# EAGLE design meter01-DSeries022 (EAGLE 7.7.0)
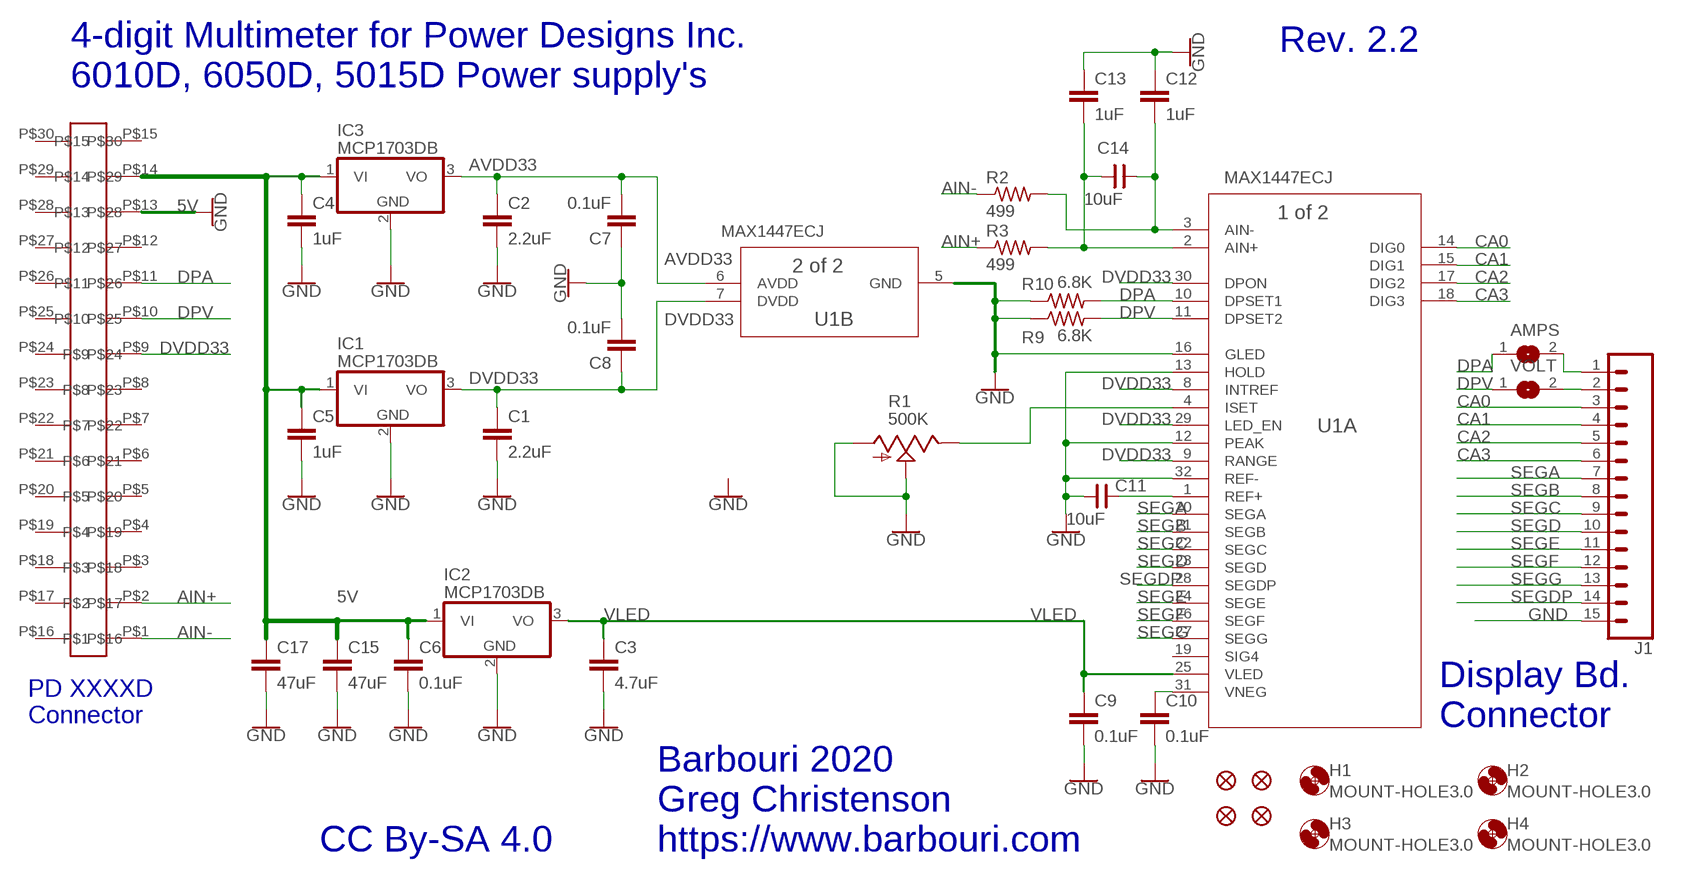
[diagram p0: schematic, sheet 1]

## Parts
AMPS  SJ  [SJ]
C1  2.2uF  2.2UF-0805-25V-(+80/-20%)  [0805]
C2  2.2uF  2.2UF-0805-25V-(+80/-20%)  [0805]
C3  4.7uF  2.2UF-0805-25V-(+80/-20%)  [0805]
C4  1uF  0.1UF-0603-25V-5%  [0603]
C5  1uF  0.1UF-0603-25V-5%  [0603]
C6  0.1uF  0.1UF-0603-25V-5%  [0603]
C7  0.1uF  0.1UF-0603-25V-5%  [0603]
C8  0.1uF  0.1UF-0603-25V-5%  [0603]
C9  0.1uF  0.1UF-0603-25V-5%  [0603]
C10  0.1uF  0.1UF-0603-25V-5%  [0603]
C11  10uF  CNP-0805  [0805]
C12  1uF  0.1UF-0603-25V-5%  [0603]
C13  1uF  0.1UF-0603-25V-5%  [0603]
C14  10uF  CNP-0805  [0805]
C15  47uF  C-EUC1206  [C1206]
C17  47uF  C-EUC1206  [C1206]
FD1  FIDUCIALUFIDUCIAL  [FIDUCIAL-MICRO]
FD2  FIDUCIALUFIDUCIAL  [FIDUCIAL-MICRO]
FD3  FIDUCIALUFIDUCIAL  [FIDUCIAL-MICRO]
FD4  FIDUCIALUFIDUCIAL  [FIDUCIAL-MICRO]
H1  MOUNT-HOLE3.0  [3,0]
H2  MOUNT-HOLE3.0  [3,0]
H3  MOUNT-HOLE3.0  [3,0]
H4  MOUNT-HOLE3.0  [3,0]
IC1  MCP1703DB  [SOT223]
IC2  MCP1703DB  [SOT223]
IC3  MCP1703DB  [SOT223]
J1  CONN_15LOCK  [1X15_LOCK]
R1  500K  TRIM_US-SM-42/43W  [SM-42/43W]
R2  499  R-US_M1206  [M1206]
R3  499  R-US_M1206  [M1206]
R9  6.8K  R-US_R0805  [R0805]
R10  6.8K  R-US_R0805  [R0805]
U1  MAX1447ECJ  MAX1447ECJ+21-0054G_32-L  [21-0054G_32-L]
U$2  EDGECARD15  [EDGECARD15]
VOLT  SJ  [SJ]

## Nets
5V: C4.1 C5.1 C6.1 C15.1 C17.1 IC1.1(VI) IC2.1(VI) IC3.1(VI) U$2.P$14
AIN+: R3.1 U$2.P$2
AIN-: R2.1 U$2.P$1
AVDD33: C2.1 C7.2 IC3.3(VO) U1.6(B:AVDD)
CA0: J1.3 U1.14(A:DIG0)
CA1: J1.4 U1.15(A:DIG1)
CA2: J1.5 U1.17(A:DIG2)
CA3: J1.6 U1.18(A:DIG3)
DPA: AMPS.1 R10.2 U1.10(A:DPSET1) U$2.P$11
DPV: R9.2 U1.11(A:DPSET2) U$2.P$10 VOLT.1
DVDD33: C1.1 C8.1 IC1.3(VO) U1.7(B:DVDD) U1.8(A:INTREF) U1.9(A:RANGE) U1.29(A:LED_EN) U1.30(A:DPON) U$2.P$9
GND: C1.2 C2.2 C3.2 C4.2 C5.2 C6.2 C7.1 C8.2 C9.2 C10.2 C11.1 C12.1 C13.1 C15.2 C17.2 IC1.2(GND) IC2.2(GND) IC3.2(GND) J1.15 R1.1(A) R1.2(S) R9.1 R10.1 U1.5(B:GND) U1.12(A:PEAK) U1.13(A:HOLD) U1.16(A:GLED) U1.32(A:REF-) U$2.P$13
N$1: C13.2 C14.1 R3.2 U1.2(A:AIN+)
N$2: C12.2 C14.2 R2.2 U1.3(A:AIN-)
N$5: AMPS.2 J1.1
N$6: J1.2 VOLT.2
N$7: R1.3(E) U1.4(A:ISET)
N$9: C10.1 U1.31(A:VNEG)
N$10: C11.2 U1.1(A:REF+)
SEGA: J1.7 U1.20(A:SEGA)
SEGB: J1.8 U1.21(A:SEGB)
SEGC: J1.9 U1.22(A:SEGC)
SEGD: J1.10 U1.23(A:SEGD)
SEGDP: J1.14 U1.28(A:SEGDP)
SEGE: J1.11 U1.24(A:SEGE)
SEGF: J1.12 U1.26(A:SEGF)
SEGG: J1.13 U1.27(A:SEGG)
VLED: C3.1 C9.1 IC2.3(VO) U1.25(A:VLED)
Unconnected: U1.19(A:SIG4) U$2.P$3 U$2.P$4 U$2.P$5 U$2.P$6 U$2.P$7 U$2.P$8 U$2.P$12 U$2.P$15 U$2.P$16 U$2.P$17 U$2.P$18 U$2.P$19 U$2.P$20 U$2.P$21 U$2.P$22 U$2.P$23 U$2.P$24 U$2.P$25 U$2.P$26 U$2.P$27 U$2.P$28 U$2.P$29 U$2.P$30

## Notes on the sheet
- Rev. 2.2
- 4-digit Multimeter for Power Designs Inc.
  6010D, 6050D, 5015D Power supply's
- PD XXXXD
  Connector
- Display Bd.
  Connector
- CC By-SA 4.0
- Barbouri 2020
  Greg Christenson
  https://www.barbouri.com

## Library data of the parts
AMPS VOLT = jumper:SJ: SMD solder JUMPER
C1 C2 = SparkFun-Capacitors:2.2UF: 2.2µF ceramic capacitors; PROD_ID: CAP-11624
C3 = SparkFun-Capacitors:2.2UF: 2.2µF ceramic capacitors; PROD_ID: CAP-11624; VALUE: 2.2uF
C4 C5 = SparkFun-Capacitors:0.1UF: 0.1µF ceramic capacitors; PROD_ID: CAP-08604; VALUE: 0.1uF
C6-C10 = SparkFun-Capacitors:0.1UF: 0.1µF ceramic capacitors; PROD_ID: CAP-08604
C11 = cap-master:CNP-: NON-POLARIZED CAP; DESC: 10µF ±10% 10V Ceramic Capacitor X7R 0805 (2012 Metric); MFG: AVX Corp; PN: 0805ZC106KAT4A
C12 C13 = SparkFun-Capacitors:0.1UF: 0.1µF ceramic capacitors; DESC: 1µF ±10% 16V Ceramic Capacitor X7R 0603 (1608 Metric); MFG: Vishay Vitramon; PN: VJ0603Y105KXJCW1BC; PROD_ID: CAP-08604; VALUE: 0.1uF
C14 = cap-master:CNP-: NON-POLARIZED CAP
C15 C17 = resistor:C-EU: CAPACITOR, European symbol; DESC: 47µF Molded Tantalum Capacitors 10V 1206 (3216 Metric) 1.5Ohm; MFG: AVX Corp; PN: TLJG476M010R1500
FD1-FD4 = SparkFun-Aesthetics:FIDUCIAL: Fiducial Alignment Points
H1-H4 = holes:MOUNT-HOLE: MOUNTING HOLE with drill center marker
IC1-IC3 = linear:MCP1703: 250 mA, 16V, Low Quiescent Current LDO Regulator Source: http://ww1.microchip.com/downloads/en/DeviceDoc/22049b.pdf
J1 = SparkFun-Connectors:CONN_15: Multi connection point. Often used as Generic Header-pin footprint for 0.1 inch spaced/style header connections On any of the 0.1 inch spaced packages, you can populate with these: Break Away Headers - Straight (PRT-00116) Break Away Male Headers - Right Angle (PRT-00553) Female Headers (PRT-00115)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
R1 = pot:TRIM_US-: POTENTIOMETER; DESC: 500 kOhms 0.25W, 1/4W J Lead Surf Mnt Trimmer Cermet 12 Turn Top Adj; MFG: Bourns Inc; PN: 3224W-1-504E
R2 R3 = resistor:R-US_: RESISTOR, American symbol; DESC: 499 Ohms ±0.1% 0.4W, 2/5W 1206 Non-Inductive Thin Film; MFG: Vishay Thin Film; PN: PTN1206Y4990BST1
R9 R10 = resistor:R-US_: RESISTOR, American symbol
U1 = MAX1447:MAX1447ECJ+; MANUFACTURER_PART_NUMBER: MAX1447ECJ+; VENDOR: Maxim Integrated Products
U$2 = User-Submitted:EDGECARD15: 15 pin edge card connector fingers 0.1" spacing 0.25" length. top and bottom layers 30 total pins

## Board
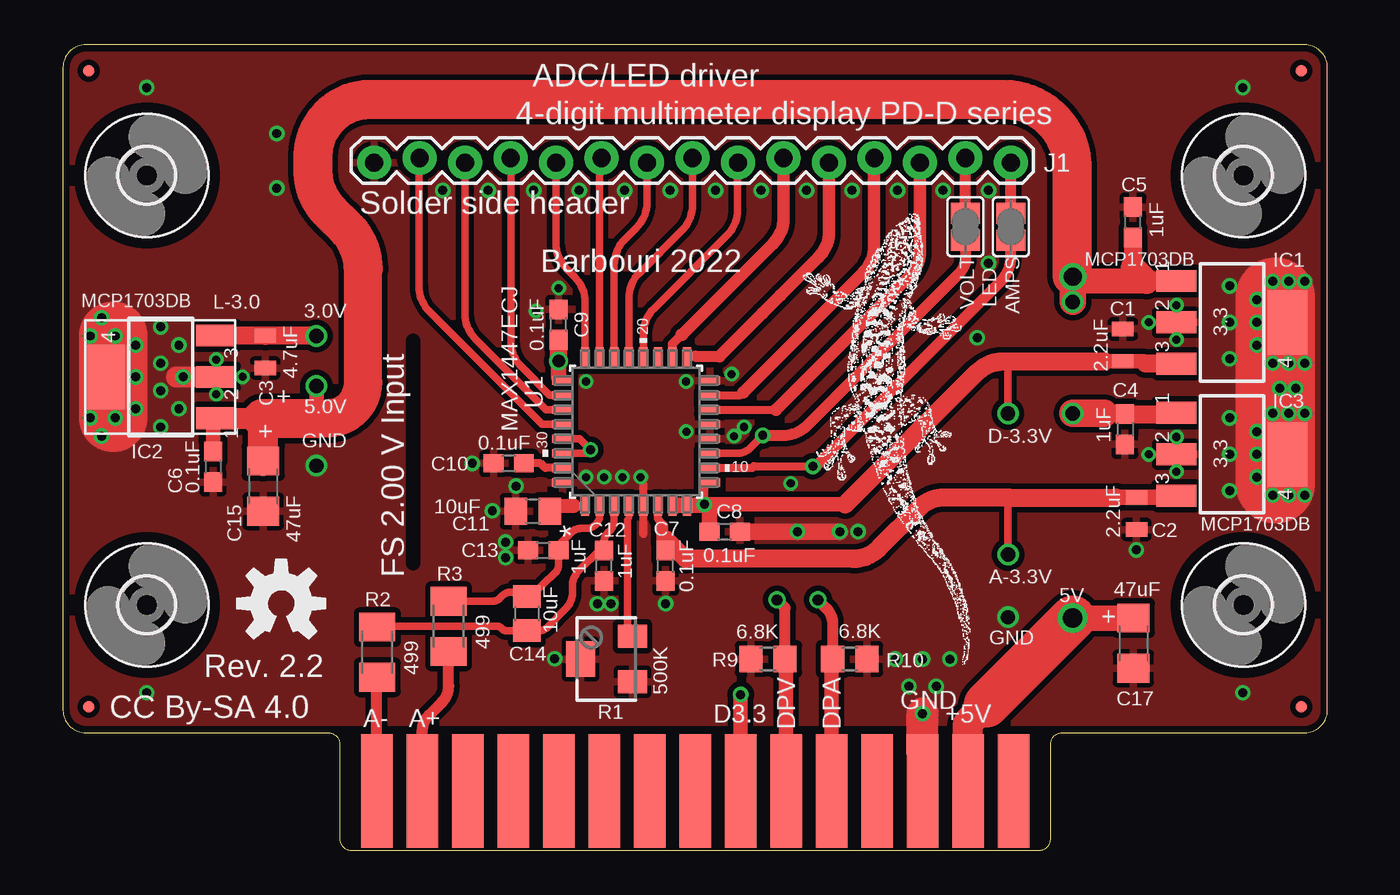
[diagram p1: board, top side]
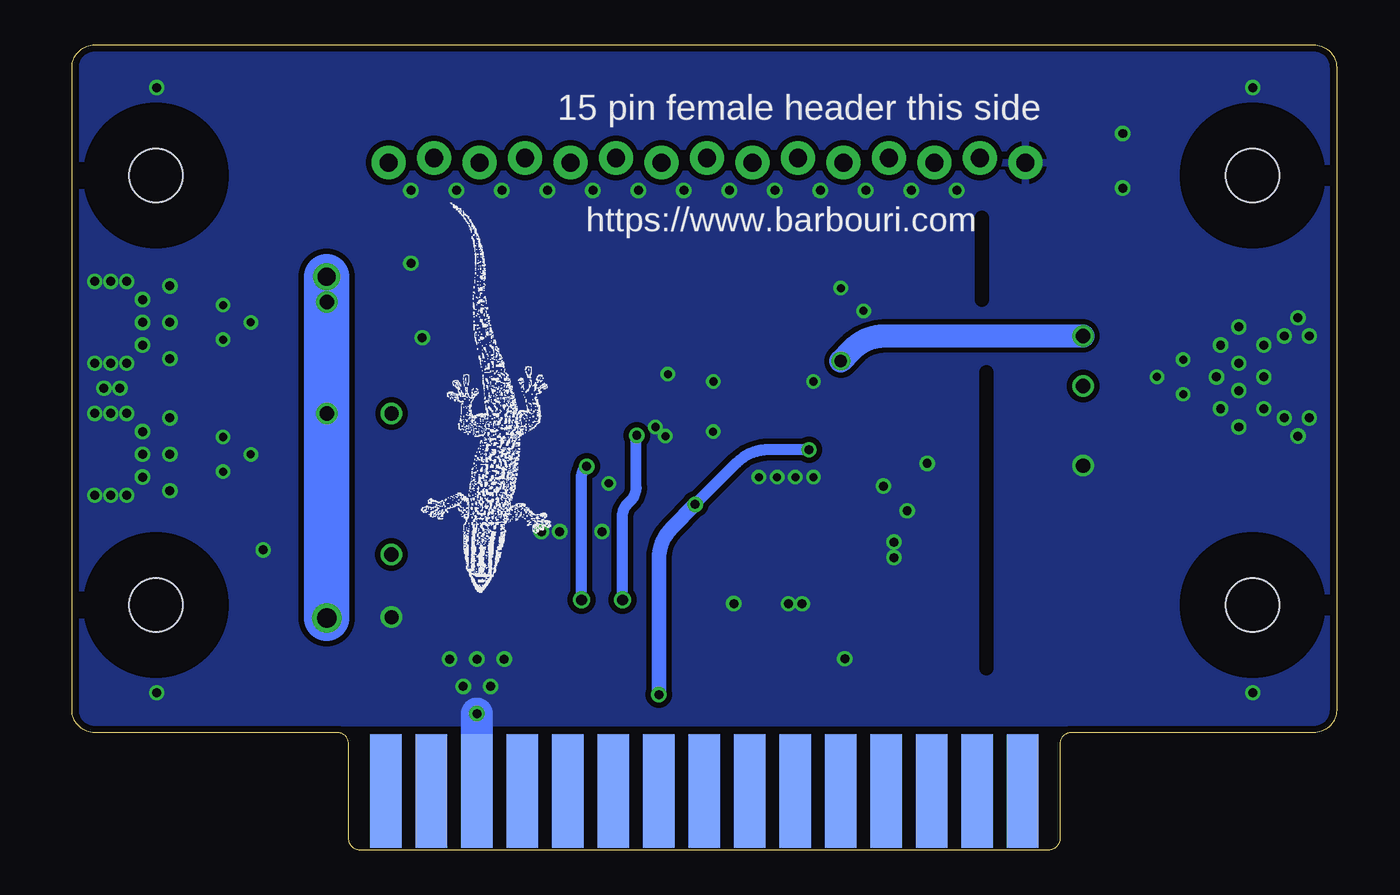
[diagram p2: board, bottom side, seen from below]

Size 70.61 x 44.96 mm. Coordinates in mm from the lower left corner, seen from the top.
Outline: 55.75,6.55 69.34,6.55 arc90 70.61,7.82 70.61,43.69 arc90 69.34,44.96 1.27,44.96 arc90 0,43.69 0,7.82 arc90 1.27,6.55 14.86,6.55 arc-90 15.44,5.92 15.44,0.64 arc90 16.13,0 54.48,0 arc90 55.17,0.64 55.17,5.92 arc-90 55.75,6.55
Copper layers (1*16): Top 0.0356mm / dielectric 1.5011mm / Bottom 0.0356mm
Design rules "oshpark-2layer *": minimum track width 16mil, minimum drill 9mil, track to track 12mil, track to pad 12mil, pad to pad 12mil, via to via 8mil, smd to smd 8mil, copper to edge 15mil, drill to drill 6mil, minimum pad ring 7mil, minimum via ring 7mil, stop-mask expansion 2.5mil, vias tented up to drill 20mil, thermal gap 10mil
tRestrict: 1 lines
bRestrict: 2 lines

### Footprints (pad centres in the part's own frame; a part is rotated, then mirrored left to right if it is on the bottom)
SJ = smd 1.168 x 1.6: 1 -0.762,0; 2 0.762,0
0805 = smd 0.8 x 1.2: 1 -0.9,0; 2 0.9,0
0603 = smd 1.1 x 1: 1 -0.85,0; 2 0.85,0
0805' = smd 1.27 x 1.524: 1 -0.953,0; 2 0.953,0
C1206 = smd 1.6 x 1.8: 1 -1.4,0; 2 1.4,0
FIDUCIAL-MICRO = smd 0.635 x 0.635: 1 0,0
3,0 = hole 3: 0,0
SOT223 = smd 1.219 x 2.235: 1 -2.311,-3.099; 2 0,-3.099; 3 2.311,-3.099 | smd 3.6 x 2.2: 4 0,3.099
1X15_LOCK = drill 1.016 pad 1.88: 1 0,0.127; 2 2.54,-0.127; 3 5.08,0.127; 4 7.62,-0.127; 5 10.16,0.127; 6 12.7,-0.127; 7 15.24,0.127; 8 17.78,-0.127; 9 20.32,0.127; 10 22.86,-0.127; 11 25.4,0.127; 12 27.94,-0.127; 13 30.48,0.127; 14 33.02,-0.127; 15 35.56,0.127
SM-42/43W = smd 1.3 x 1.6: 1 -1.27,-1.45; 3 1.27,-1.45 | smd 2 x 1.6: 2 0,1.45
M1206 = smd 1.6 x 2: 1 -1.4,0; 2 1.4,0
R0805 = smd 1.3 x 1.5: 1 -0.95,0; 2 0.95,0
21-0054G_32-L = smd 1.168 x 0.457: 1 -4.115,2.845; 2 -4.115,2.032; 3 -4.115,1.219; 4 -4.115,0.406; 5 -4.115,-0.406; 6 -4.115,-1.219; 7 -4.115,-2.032; 8 -4.115,-2.845; 17 4.115,-2.845; 18 4.115,-2.032; 19 4.115,-1.219; 20 4.115,-0.406; 21 4.115,0.406; 22 4.115,1.219; 23 4.115,2.032; 24 4.115,2.845 | smd 0.457 x 1.168: 9 -2.845,-4.115; 10 -2.032,-4.115; 11 -1.219,-4.115; 12 -0.406,-4.115; 13 0.406,-4.115; 14 1.219,-4.115; 15 2.032,-4.115; 16 2.845,-4.115; 25 2.845,4.115; 26 2.032,4.115; 27 1.219,4.115; 28 0.406,4.115; 29 -0.406,4.115; 30 -1.219,4.115; 31 -2.032,4.115; 32 -2.845,4.115
EDGECARD15 = smd 1.778 x 6.35: P$1 -17.78,3.302; P$2 -15.24,3.302; P$3 -12.7,3.302; P$4 -10.16,3.302; P$5 -7.62,3.302; P$6 -5.08,3.302; P$7 -2.54,3.302; P$8 0,3.302; P$9 2.54,3.302; P$10 5.08,3.302; P$11 7.62,3.302; P$12 10.16,3.302; P$13 12.7,3.302; P$14 15.24,3.302; P$15 17.78,3.302 | smd 1.778 x 6.35 bottom: P$16 -17.78,3.302; P$17 -15.24,3.302; P$18 -12.7,3.302; P$19 -10.16,3.302; P$20 -7.62,3.302; P$21 -5.08,3.302; P$22 -2.54,3.302; P$23 0,3.302; P$24 2.54,3.302; P$25 5.08,3.302; P$26 7.62,3.302; P$27 10.16,3.302; P$28 12.7,3.302; P$29 15.24,3.302; P$30 17.78,3.302

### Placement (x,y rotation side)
AMPS  52.93,34.8 90 top
C1  59.18,28.19 90 top
C2  59.94,18.8 270 top
C3  11.3,27.81 270 top
C4  59.31,23.5 270 top
C5  59.75,35.05 90 top
C6  8.38,21.4 270 top
C7  33.66,15.88 90 top
C8  36.96,17.78 0 top
C9  27.69,29.34 90 top
C10  24.89,21.59 180 top
C11  10uF  [0805']  26.24,18.92 0 top
C12  30.23,15.88 90 top
C13  26.82,16.74 0 top
C14  10uF  [0805']  25.91,13.21 270 top
C15  11.18,20.32 270 top
C17  59.78,11.56 270 top
FD1  69.16,8 90 top
FD2  1.45,8 90 top
FD3  69.16,43.51 90 top
FD4  1.45,43.51 90 top
H1  4.69,13.69 0 top
H2  65.93,13.69 0 top
H3  4.69,37.67 0 top
H4  65.93,37.67 0 top
IC1  65.28,29.46 270 top
IC2  5.46,26.42 90 top
IC3  65.28,22.1 270 top
J1  52.93,38.51 180 top
R1  30.35,10.67 90 top
R2  17.55,11.05 90 top
R3  21.54,12.5 90 top
R9  39.37,10.67 0 top
R10  43.94,10.67 180 top
U1  32,23.37 90 top
U$1  [OSHW-LOGO-M]  12.19,13.77 0 top
U$2  35.31,0 0 top
VOLT  50.39,34.8 90 top

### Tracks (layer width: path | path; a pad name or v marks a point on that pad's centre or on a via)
5V  (via drill 0.8, 1, 1.1)
  Top 0.61: 8.38,23.68 arc-45 IC2.1
  Top 0.813: 62.12,24.34 IC3.1 | v14.16,25.91 14.15,24.11 | C6.1 8.38,23.68
  Top 1.016: 62.12,24.34 C4.1 59.52,24.38 58.17,24.38 | IC1.1 60.54,31.77 | 60.54,31.77 60.52,31.75 | 60.54,31.77 60.48,31.77 | 59.77,32.49 59.77,34.19 C5.1
  Top 1.168: IC2.1 11.15,24.11
  Top 1.27: 56.45,31.75 v56.39,32 | v56.39,12.96 v56.39,12.95
  Top 1.397: 60.52,31.75 56.45,31.75 | 60.48,31.77 59.77,32.49
  Top 1.422: C17.1 v56.39,12.96
  Top 1.473: v56.39,30.61 v56.39,32
  Top 1.524: v56.39,24.38 58.17,24.38
  Top 1.676: U$2.P$14 50.55,7.11 51.56,8.13 | 14.15,24.11 14.2,24.11 | C15.1 11.18,24.04 arc45 11.15,24.11
  Top 1.93: 14.2,24.11 14.76,24.11 | 56.35,32.04 v56.39,32
  Top 2.134: 14.76,24.11 arc90 16.76,26.11 16.76,32.47
  Top 2.184: 11.15,24.11 14.15,24.11 | 16.76,32.47 arc45 15.83,34.71 14.9,35.65 arc-45 13.97,37.89 13.97,38.73 arc-90 17.14,41.91 52.54,41.91 arc-90 56.35,38.1 56.35,32.04
  Top 2.54: 51.56,8.13 v56.39,12.95
  Bottom 2.54: v56.39,12.95 v56.39,24.38 v56.39,32
AIN+
  Top 0.61: U$2.P$2 20.07,6.64 arc-45 20.44,7.54 21.17,8.26 arc45 21.54,9.16 R3.1
AIN-
  Top 0.61: U$2.P$1 17.53,9.12 R2.1
AVDD33  (via drill 0.8)
  Top 0.406: v52.78,16.51 52.76,16.54 52.76,19.63 52.78,19.63 52.83,19.68
  Top 0.457: 33.48,18.09 33.45,18.19 33.22,18.52 U1.6
  Top 0.61: 33.66,17.37 33.55,17.35 33.48,17.17
  Top 0.66: 33.48,17.17 33.48,18.09
  Top 0.813: 62.09,19.7 IC3.3 | 58.8,19.68 57.04,19.7
  Top 0.864: C7.2 33.66,17.37 | 62.09,19.7 C2.1 57.04,19.7
  Top 0.991: 34.77,16.26 33.66,17.37
  Top 1.016: 34.77,16.26 44.13,16.26 arc45 45.54,16.84 47.8,19.1 arc-45 49.22,19.68 52.83,19.68 58.8,19.68
CA0
  Top 0.457: U1.14 39.83,24.59
  Top 0.711: 39.83,24.59 47.27,32.03 arc45 47.85,33.44 J1.3
CA1
  Top 0.457: U1.15 37.85,25.4 38,25.55
  Top 0.711: 38,25.55 44.7,32.26 arc45 45.29,33.67 45.29,38.61 J1.4
CA2
  Top 0.508: 35.3,27.58 34.87,27.5 U1.17
  Top 0.61: 35.3,27.58 36.66,27.58
  Top 0.711: 36.66,27.58 39.05,29.97 40.08,30.99 42.19,33.09 arc45 42.77,34.51 J1.5
CA3
  Top 0.508: U1.18 34.04,28.26 34.54,28.77
  Top 0.711: 34.54,28.77 34.56,28.77 39.65,33.86 arc45 40.23,35.27 J1.6
DPA  (via drill 0.5, 0.6)
  Top 0.457: U1.10 38.48,21.34 38.58,21.44 41.86,21.44 v41.87,21.43
  Top 0.61: R10.2 42.99,12.62 arc45 42.62,13.51 v42.16,13.97 | v41.87,21.43 42.05,21.43 52.35,31.72 arc45 52.93,33.14 AMPS.1
  Top 0.813: U$2.P$11 42.93,10.6 R10.2
  Bottom 0.61: v42.16,13.97 42.16,20.87 arc45 41.98,21.32 v41.87,21.43
DPV  (via drill 0.5, 0.6)
  Top 0.432: U1.11 37.66,22.15 arc45 38.37,22.44 v39.08,23.15
  Top 0.61: R9.2 40.32,13.53 v39.88,13.97 | v39.08,23.15 40.18,23.15 arc45 41.59,23.74 50.05,32.19 arc45 50.42,33.09 50.42,34.01 VOLT.1
  Top 0.813: U$2.P$10 40.39,10.6 R9.2
  Bottom 0.61: v39.88,13.97 39.88,18.64 arc45 39.59,19.34 39.41,19.52 arc-45 39.12,20.23 39.12,23.11 v39.08,23.15
DVDD33  (via drill 0.5, 0.8)
  Top 0.406: 34.89,19.21 U1.8 U1.7 | v52.77,24.38 52.77,27.22 52.83,27.28 | U1.29 28.85,22.96 v29.46,22.35 29.26,22.15 U1.30 | U1.9 35.81,20.52 v35.81,19.3
  Top 0.457: U1.7 34.24,19.25
  Top 0.762: 60.34,27.29 60.45,27.18
  Top 0.813: 43.69,19.3 v35.81,19.3 | U$2.P$9 v37.85,8.69 | 60.34,27.29 C1.1 59.17,27.28 58.17,27.28
  Top 0.864: C8.1 36.11,19.01 v35.81,19.3 35.76,19.25 U1.8 34.24,19.25
  Top 1.016: 43.69,19.3 51.08,26.69 arc-45 52.49,27.28 52.83,27.28 58.17,27.28 | 60.45,27.18 62.15,27.18 IC1.3
  Bottom 0.61: v29.46,22.35 31.73,22.35 arc-45 33.5,21.62 v35.81,19.3
  Bottom 0.813: v37.85,8.69 37.85,16.24 arc45 37.11,18 v35.81,19.3
GND  (via drill 0.45, 0.5, 0.8)
  Top 0.457: 32.41,17.65 32.41,20.45 | 2.79,24.13 v2.92,24.13 | 48.01,5.33 U$2.P$13 | 67.69,20.45 67.69,19.94 v67.56,19.81
  Top 0.914: 38.1,17.78 v43.38,17.78
  Top 1.168: 6.35,26.42 7.87,26.42
  Top 1.778: 48.01,5.33 v48.01,7.62
  Top 3.81: 2.79,24.13 2.79,28.7
  Top 4.445: 67.69,20.45 67.69,30.86
  Bottom 1.778: 48.01,5.33 v48.01,7.62
  other vias: 27.69,31.37 26.42,30.1 33.66,13.77 38.04,23.62 37.34,26.57 40.64,20.47 1.52,24.13 1.52,28.7 2.92,28.7 4.06,24.64 4.06,28.19 4.06,26.42 6.71,26.42 6.48,24.64 10.03,26.42 8.56,25.45 8.56,27.38 6.48,28.19 67.56,27.18 68.45,27.18 69.34,27.18 67.94,25.78 68.83,25.78 66.67,22.1 66.67,29.46 66.67,28.19 66.67,30.73 68.45,19.81 69.34,19.81 66.67,20.83 66.67,23.37 67.56,24.38 68.45,24.38 69.34,24.38 67.56,31.75 68.45,31.75 69.34,31.75 65.15,29.46 65.15,27.43 65.15,31.5 65.15,22.1 65.15,20.07 65.15,24.13 62.18,21.13 62.18,23.06 62.18,28.5 62.18,30.43 60.63,22.1 60.63,29.46 34.8,26.16 32.26,20.83 23.98,18.95 24.71,17.2 11.94,40.01 29.21,20.83 22.86,21.59 30.61,13.75 14.16,21.46 29.21,26.16 30.23,20.83 31.24,20.83 59.94,16.76 51.69,32.77 2.16,23.11 2.16,29.72 11.94,36.96 5.46,25.65 5.46,27.18 5.46,29.21 5.46,23.62 46.61,36.83 44.07,36.83 41.53,36.83 38.99,36.83 36.45,36.83 33.91,36.83 28.83,36.83 26.29,36.83 49.15,36.83 31.37,36.83 23.75,36.83 21.21,36.83 34.81,23.37 51.05,28.6 52.77,13 4.67,42.57 4.67,8.79 65.89,8.79 65.89,42.57 48.01,10.67 24.71,16.33 29.84,13.75 44.4,17.78 51.69,36.83 41.02,17.78 25.3,20.32 27.46,10.68 49.53,10.67 46.48,10.67 37.48,23.11 47.24,9.14 48.77,9.14
  pour Top: 70.61,7.14 0,7.14 0,44.96 70.61,44.96
  pour Bottom: 70.61,7.11 0,7.11 0,44.96 70.61,44.96
N$1
  Top 0.406: U1.2 29.97,18.68 arc-45 29.79,18.23 29.7,18.14 arc-45 29.25,17.96 28.89,17.96 arc45 28.44,17.77 27.69,17.02 27.69,16.75 C13.2 27.67,15.93 arc-45 27.49,15.48 26.16,14.22 26.16,14.41 C14.1 25.89,14.4 25,14.4 arc45 24.55,14.22 24.42,14.08 arc-45 23.97,13.9 R3.2
N$2
  Top 0.406: U1.3 30.79,18.35 arc-45 30.6,17.9 30.41,17.71 arc45 30.23,17.26 C12.2 29.93,16.73 28.82,15.61 arc45 28.45,14.71 28.45,14.37 arc-45 28.08,13.47 27.03,12.43 arc-45 26.59,12.24 25.92,12.24 | 25.92,12.24 C14.2 | 25.92,12.24 24.77,12.24 arc-45 24.55,12.34 24.48,12.4 arc45 24.25,12.5 17.5,12.5 R2.2
N$5
  Top 0.61: AMPS.2 J1.1
N$6
  Top 0.61: VOLT.2 J1.2
N$7
  Top 0.356: U1.4 31.6,18.54 31.53,18.41
  Top 0.406: 31.53,18.41 31.53,12.18
  Top 0.457: 31.53,12.18 31.56,12.18 R1.3
N$9
  Top 0.457: U1.31 26.92,21.34 26.67,21.59 C10.1
N$10
  Top 0.406: 27.43,19.21 27.27,19.05 C11.2 | 28.51,19.21 28.62,19.21 29.02,19.21 U1.1
  Top 0.813: 28.51,19.21 27.43,19.21
SEGA
  Top 0.406: U1.20 32.41,28.81 arc-45 33,30.23 37.08,34.31 arc45 37.67,35.73 37.67,38.35 J1.7
SEGB
  Top 0.406: U1.21 31.6,30.8 arc-45 32.18,32.21 34.57,34.59 arc45 35.15,36.01 J1.8
SEGC
  Top 0.406: U1.22 30.79,32.67 arc-45 31.37,34.09 32.03,34.75 arc45 32.61,36.16 J1.9
SEGD
  Top 0.406: U1.23 29.97,38.53 J1.10
SEGDP
  Top 0.406: U1.28 26.75,23.77 20.47,30.05 arc-45 19.89,31.46 19.89,38.61 J1.14
SEGE
  Top 0.406: U1.24 29.16,30.59 arc45 28.57,32.01 28.12,32.46 arc-45 27.53,33.87 J1.11
SEGF
  Top 0.406: U1.26 27.18,25.4 25.61,26.97 arc-45 25.02,28.39 25.02,38.61 J1.12
SEGG
  Top 0.406: U1.27 26.98,24.59 23.04,28.52 arc-45 22.45,29.94 J1.13
VLED  (via drill 0.7, 0.8)
  Top 0.406: 27.75,26.19 U1.25 | 8.54,28.64 IC2.3
  Top 0.508: U1.25 27.69,26.42
  Top 0.813: 8.62,28.71 8.54,28.64 | 11.31,28.7 C3.1
  Top 0.864: 27.69,26.42 v27.69,27.3
  Top 0.965: C9.1 v27.69,27.3
  Top 1.016: 8.38,28.78 IC2.3 | C3.1 8.62,28.71 | v14.16,28.7 11.31,28.7
  Bottom 1.27: v27.69,27.3 27.02,27.97 arc45 25.25,28.7 v14.16,28.7

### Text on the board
tNames: ADC/LED driver | 4-digit multimeter display PD-D series | Solder side header | LED | Barbouri 2022 | L-3.0 | 3.0V | 20 | 3.3 | + | 5.0V | D-3.3V | + | GND | 30 | 10 | 3.3 | A-3.3V | FS 2.00 V Input | 5V | + | GND | Rev. 2.2 | DPV | DPA | GND | CC By-SA 4.0 | A- | A+ | D3.3 | +5V
bNames: 15 pin female header this side | https://www.barbouri.com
